PROGRAM MAIN
VAR
	p07_ST_motor_0: p07_ST_motor;
	tipkaLevo: BOOL;
	tipkaDesno: BOOL;
	motorPremik: BOOL;
	motorSmer: BOOL;
	FB_spremljanjeMateriala: p08_ST_spremljanjeMateriala;
END_VAR

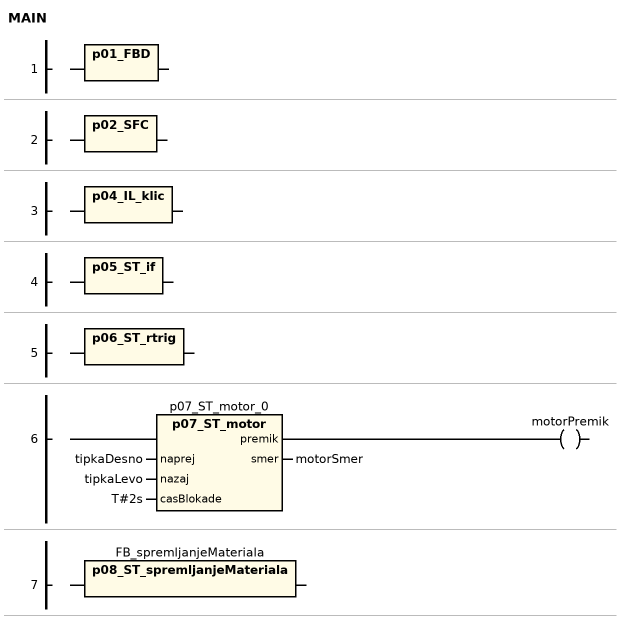
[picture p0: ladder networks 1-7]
// NETWORK 1
p01_FBD();

// NETWORK 2
p02_SFC();

// NETWORK 3
p04_IL_klic();

// NETWORK 4
p05_ST_if();

// NETWORK 5
p06_ST_rtrig();

// NETWORK 6
p07_ST_motor_0(naprej := tipkaDesno, nazaj := tipkaLevo, casBlokade := T#2s, smer => motorSmer); // p07_ST_motor
motorPremik := p07_ST_motor_0.premik;

// NETWORK 7
FB_spremljanjeMateriala(); // p08_ST_spremljanjeMateriala

END_PROGRAM
